[IBIS Ver]   3.2
[File Name]   sprm298.ibs
[File Rev]   1.0
[Date]   November 3, 2003
[Source]   File originated at Texas Instruments
[Copyright]   (c) 2003, Texas Instruments Inc.
[Component]   f2812pgf
[Manufacturer] Texas Instruments
[Package]
| Variable   Typ   Min   Max
R_pkg   0.198   0.1909   0.2047
L_pkg   8.904e-09   8.346e-09   9.905e-09
C_pkg   1.561e-12   1.156e-12   1.834e-12
[Pin] signal_name   model_name   R_pin   L_pin   C_pin
1   VDDAIO   NC   0.1921  9.905e-09  1.489e-12
2   ADCINB0   ioh125   0.1951  9.662e-09  1.834e-12
3   ADCINB1   ioh125   0.198   9.558e-09  1.805e-12
4   ADCINB2   ioh125   0.2006  9.473e-09  1.771e-12
5   ADCINB3   ioh125   0.2031  9.41e-09   1.706e-12
6   ADCINB4   ioh125   0.2036  9.308e-09  1.669e-12
7   ADCINB5   ioh125   0.2017  9.182e-09  1.673e-12
8   ADCINB6   ioh125   0.2002  9.071e-09  1.647e-12
9   ADCINB7   ioh125   0.1989  8.977e-09  1.625e-12
10   ADCREFM   ioh125   0.1977  8.88e-09   1.606e-12
11   ADCREFP   ioh125   0.1967  8.794e-09  1.581e-12
12   AVSSREFBG   ioh125   0.1961  8.721e-09  1.56e-12
13   AVDDREFBG   ioh125   0.1955  8.646e-09  1.544e-12
14   VDDA1   NC   0.195   8.579e-09  1.521e-12
15   VSSA1   NC   0.1949  8.524e-09  1.503e-12
16   ADCRESEXT   ioh125   0.1948  8.469e-09  1.489e-12
17   XMPNMC   idg095_pe1005   0.1948  8.424e-09  1.468e-12
18   XA(0)   oui835   0.1952  8.388e-09  1.452e-12
19   VSS   NC   0.1954  8.359e-09  1.442e-12
20   MDRA   idg095_ouo435_ps1005  0.196   8.346e-09  1.424e-12
21   XD(0)   idg095_oui835_ps1005  0.1967  8.36e-09   1.411e-12
22   MDXA   idg095_ouo435   0.1975  8.421e-09  1.16e-12
23   VDD   NC   0.198   8.429e-09  1.156e-12
24   XD(1)   idg095_oui835_ps1005  0.1973  8.376e-09  1.412e-12
25   MCLKRA   idg095_ouo435_ps1005  0.1971  8.373e-09  1.43e-12
26   MFSXA   idg095_ouo435_ps1005  0.197   8.398e-09  1.442e-12
27   XD(2)   idg095_oui835_ps1005  0.197   8.435e-09  1.457e-12
28   MCLKXA   idg095_ouo435_ps1005  0.1974  8.484e-09  1.476e-12
29   MFSRA   idg095_ouo435_ps1005  0.1977  8.542e-09  1.493e-12
30   XD(3)   idg095_oui835_ps1005  0.1984  8.61e-09   1.5e-12
31   VDDIO   NC   0.1982  8.656e-09  1.517e-12
32   VSS   NC   0.1989  8.731e-09  1.548e-12
33   XD(4)   idg095_oui835_ps1005  0.2001  8.817e-09  1.558e-12
34   SPICLKA   idg095_ouo435   0.1999  8.873e-09  1.577e-12
35   SPISTEA   idg095_ouo435   0.2013  8.967e-09  1.609e-12
36   XD(5)   idg095_oui835_ps1005  0.2027  9.071e-09  1.622e-12
37   VDD   NC   0.2027  9.139e-09  1.641e-12
38   VSS   NC   0.2047  9.255e-09  1.665e-12
39   XD(6)   idg095_oui835_ps1005  0.2047  9.341e-09  1.652e-12
40   SPISIMOA   idg095_ouo435   0.2031  9.409e-09  1.689e-12
41   SPISOMIA   idg095_ouo435   0.1983  9.422e-09  1.757e-12
42   XRDn   oui835   0.1956  9.501e-09  1.801e-12
43   XA(1)   oui835   0.1933  9.619e-09  1.832e-12
44   XZCS0AND1n   oui835   0.1909  9.876e-09  1.489e-12
45   PWM7   sw0145_ouo435_ups285  0.1921  9.905e-09  1.489e-12
46   PWM8   sw0145_ouo435_ups285  0.1951  9.662e-09  1.834e-12
47   PWM9   sw0145_ouo435_ups285  0.198   9.558e-09  1.805e-12
48   PWM10   sw0145_ouo435_ups285  0.2006  9.473e-09  1.771e-12
49   PWM11   sw0145_ouo435_ups285  0.2031  9.41e-09   1.706e-12
50   PWM12   sw0145_ouo435_ups285  0.2036  9.308e-09  1.669e-12
51   XRNW   oui835   0.2017  9.182e-09  1.673e-12
52   VSS   NC   0.2002  9.071e-09  1.647e-12
53   T3PWM_T3CMP   sw0145_ouo435_ups285  0.1989  8.977e-09  1.625e-12
54   XD(7)   idg095_oui835_ps1005  0.1977  8.88e-09   1.606e-12
55   T4PWM_T4CMP   sw0145_ouo435_ups285  0.1967  8.794e-09  1.581e-12
56   VDD   NC   0.1961  8.721e-09  1.56e-12
57   CAP4_QEP3   sw0145_ouo435_ups285  0.1955  8.646e-09  1.544e-12
58   VSS   NC   0.195   8.579e-09  1.521e-12
59   CAP5_QEP4   sw0145_ouo435_ups285  0.1949  8.524e-09  1.503e-12
60   CAP6_QEPI2   sw0145_ouo435_ups285  0.1948  8.469e-09  1.489e-12
61   C4TRIPn   sw0145_ouo435_ups285  0.1948  8.424e-09  1.468e-12
62   C5TRIPn   sw0145_ouo435_ups285  0.1952  8.388e-09  1.452e-12
63   C6TRIPn   sw0145_ouo435_ups285  0.1954  8.359e-09  1.442e-12
64   VDDIO   NC   0.196   8.346e-09  1.424e-12
65   XD(8)   idg095_oui835_ps1005  0.1967  8.36e-09   1.411e-12
66   TEST2   iog195   0.1975  8.421e-09  1.16e-12
67   TEST1   iog195   0.198   8.429e-09  1.156e-12
68   XD(9)   idg095_oui835_ps1005  0.1973  8.376e-09  1.412e-12
69   VDD3VFL   NC   0.1971  8.373e-09  1.43e-12
70   VSS   NC   0.197   8.398e-09  1.442e-12
71   TDIRB   sw0145_ouo435_ups285  0.197   8.435e-09  1.457e-12
72   TCLKINB   sw0145_ouo435_ups285  0.1974  8.484e-09  1.476e-12
73   XD(10)   idg095_oui835_ps1005  0.1977  8.542e-09  1.493e-12
74   XD(11)   idg095_oui835_ps1005  0.1984  8.61e-09   1.5e-12
75   VDD   NC   0.1982  8.656e-09  1.517e-12
76   X2   NC   0.1989  8.731e-09  1.548e-12
77   X1/XCLKIN   NC   0.2001  8.817e-09  1.558e-12
78   VSS   NC   0.1999  8.873e-09  1.577e-12
79   T3CTRIP_PDPINTBn idg095_ouo435_ps1005  0.2013  8.967e-09  1.609e-12
80   XA(2)   oui835   0.2027  9.071e-09  1.622e-12
81   VDDIO   NC   0.2027  9.139e-09  1.641e-12
82   XHOLDAn   oui835   0.2047  9.255e-09  1.665e-12
83   T4CTRIPn/EVBSOCn idg095_ouo435_ps1005  0.2047  9.341e-09  1.652e-12
84   XWEn   oui835   0.2031  9.409e-09  1.689e-12
85   XA(3)   oui835   0.1983  9.422e-09  1.757e-12
86   VSS   NC   0.1956  9.501e-09  1.801e-12
87   CANTXA   idg095_ouo435_ps1005  0.1933  9.619e-09  1.832e-12
88   XZCS2n   oui835   0.1909  9.876e-09  1.489e-12
89   CANRXA   idg095_ouo435_ps1005  0.1921  9.905e-09  1.489e-12
90   SCITXDB   idg095_ouo435   0.1951  9.662e-09  1.834e-12
91   SCIRXDB   idg095_ouo435   0.198   9.558e-09  1.805e-12
92   PWM1   idg095_ouo435_ps1005  0.2006  9.473e-09  1.771e-12
93   PWM2   idg095_ouo435_ps1005  0.2031  9.41e-09   1.706e-12
94   PWM3   idg095_ouo435_ps1005  0.2036  9.308e-09  1.669e-12
95   PWM4   idg095_ouo435_ps1005  0.2017  9.182e-09  1.673e-12
96   XD(12)   idg095_oui835_ps1005  0.2002  9.071e-09  1.647e-12
97   XD(13)   idg095_oui835_ps1005  0.1989  8.977e-09  1.625e-12
98   PWM5   idg095_ouo435_ps1005  0.1977  8.88e-09   1.606e-12
99   VSS   NC   0.1967  8.794e-09  1.581e-12
100   VDD   NC   0.1961  8.721e-09  1.56e-12
101   PWM6   idg095_ouo435_ps1005  0.1955  8.646e-09  1.544e-12
102   T1PWM_T1CMP   idg095_ouo435_ps1005  0.195   8.579e-09  1.521e-12
103   XA(4)   oui835   0.1949  8.524e-09  1.503e-12
104   T2PWM_T2CMP   idg095_ouo435_ps1005  0.1948  8.469e-09  1.489e-12
105   VSS   NC   0.1948  8.424e-09  1.468e-12
106   CAP1_QEP1   idg095_ouo435_ps1005  0.1952  8.388e-09  1.452e-12
107   CAP2_QEP2   idg095_ouo435_ps1005  0.1954  8.359e-09  1.442e-12
108   XA(5)   oui835   0.196   8.346e-09  1.424e-12
109   CAP3_QEPI1   idg095_ouo435_ps1005  0.1967  8.36e-09   1.411e-12
110   T1CTRIP_PDPINTAn idg095_ouo435_ps1005  0.1975  8.421e-09  1.16e-12
111   XA(6)   oui835   0.198   8.429e-09  1.156e-12
112   VDD   NC   0.1973  8.376e-09  1.412e-12
113   VSS   NC   0.1971  8.373e-09  1.43e-12
114   VDDIO   NC   0.197   8.398e-09  1.442e-12
115   T2CTRIPn/EVASOCn idg095_ouo435_ps1005  0.197   8.435e-09  1.457e-12
116   TDIRA   idg095_ouo435_ps1005  0.1974  8.484e-09  1.476e-12
117   TCLKINA   idg095_ouo435_ps1005  0.1977  8.542e-09  1.493e-12
118   XA(7)   oui835   0.1984  8.61e-09   1.5e-12
119   XCLKOUT   oui835   0.1982  8.656e-09  1.517e-12
120   VSS   NC   0.1989  8.731e-09  1.548e-12
121   XA(8)   oui835   0.2001  8.817e-09  1.558e-12
122   C1TRIPn   idg095_ouo435_ps1005  0.1999  8.873e-09  1.577e-12
123   C2TRIPn   idg095_ouo435_ps1005  0.2013  8.967e-09  1.609e-12
124   C3TRIPn   idg095_ouo435_ps1005  0.2027  9.071e-09  1.622e-12
125   XA(9)   oui835   0.2027  9.139e-09  1.641e-12
126   TMS   idg095_ps1005   0.2047  9.255e-09  1.665e-12
127   TDO   oui835   0.2047  9.341e-09  1.652e-12
128   VDD   NC   0.2031  9.409e-09  1.689e-12
129   VSS   NC   0.1983  9.422e-09  1.757e-12
130   XA(10)   oui835   0.1956  9.501e-09  1.801e-12
131   TDI   idg095_ps1005   0.1933  9.619e-09  1.832e-12
132   XA(11)   oui835   0.1909  9.876e-09  1.489e-12
133   XZCS6AND7n   oui835   0.1921  9.905e-09  1.489e-12
134   TESTSEL   idg095_pe1005   0.1951  9.662e-09  1.834e-12
135   TRSTn   idg095_pe1005   0.198   9.558e-09  1.805e-12
136   TCK   idg095_ps1005   0.2006  9.473e-09  1.771e-12
137   EMU0   idg095_oui835_ps1005  0.2031  9.41e-09   1.706e-12
138   XA(12)   oui835   0.2036  9.308e-09  1.669e-12
139   XD(14)   idg095_oui835_ps1005  0.2017  9.182e-09  1.673e-12
140   XF_XPLLDIS   idg095_oui835_ps1005  0.2002  9.071e-09  1.647e-12
141   XA(13)   oui835   0.1989  8.977e-09  1.625e-12
142   VSS   NC   0.1977  8.88e-09   1.606e-12
143   VDD   NC   0.1967  8.794e-09  1.581e-12
144   XA(14)   oui835   0.1961  8.721e-09  1.56e-12
145   VDDIO   NC   0.1955  8.646e-09  1.544e-12
146   EMU1   idg095_oui835_ps1005  0.195   8.579e-09  1.521e-12
147   XD(15)   idg095_oui835_ps1005  0.1949  8.524e-09  1.503e-12
148   XA(15)   oui835   0.1948  8.469e-09  1.489e-12
149   XINT1_XBIOn   idg095_ouo435   0.1948  8.424e-09  1.468e-12
150   XNMI_XINT13   idg095_ouo435_ps1005  0.1952  8.388e-09  1.452e-12
151   XINT2_ADCSOC   idg095_ouo435   0.1954  8.359e-09  1.442e-12
152   XA(16)   oui835   0.196   8.346e-09  1.424e-12
153   VSS   NC   0.1967  8.36e-09   1.411e-12
154   VDD   NC   0.1975  8.421e-09  1.16e-12
155   SCITXDA   idg095_ouo435_ps1005  0.198   8.429e-09  1.156e-12
156   XA(17)   oui835   0.1973  8.376e-09  1.412e-12
157   SCIRXDA   idg095_ouo435_ps1005  0.1971  8.373e-09  1.43e-12
158   XA(18)   oui835   0.197   8.398e-09  1.442e-12
159   XHOLDn   idg095_ps1005   0.197   8.435e-09  1.457e-12
160   XRSn   idg095_oum425_ps1005  0.1974  8.484e-09  1.476e-12
161   XREADY   idg095_ps1005   0.1977  8.542e-09  1.493e-12
162   VDD1   NC   0.1984  8.61e-09   1.5e-12
163   VSS1   NC   0.1982  8.656e-09  1.517e-12
164   ADCBGREFIN   ioh125   0.1989  8.731e-09  1.548e-12
165   VSSA2   NC   0.2001  8.817e-09  1.558e-12
166   VDDA2   NC   0.1999  8.873e-09  1.577e-12
167   ADCINA7   ioh125   0.2013  8.967e-09  1.609e-12
168   ADCINA6   ioh125   0.2027  9.071e-09  1.622e-12
169   ADCINA5   ioh125   0.2027  9.139e-09  1.641e-12
170   ADCINA4   ioh125   0.2047  9.255e-09  1.665e-12
171   ADCINA3   ioh125   0.2047  9.341e-09  1.652e-12
172   ADCINA2   ioh125   0.2031  9.409e-09  1.689e-12
173   ADCINA1   ioh125   0.1983  9.422e-09  1.757e-12
174   ADCINA0   ioh125   0.1956  9.501e-09  1.801e-12
175   ADCLO   ioh125   0.1933  9.619e-09  1.832e-12
176   VSSAIO   NC   0.1909  9.876e-09  1.489e-12
| End of package information
| Component idg095
[Component]   idg095
[Manufacturer]   Texas Instruments
[Package]
|   typ   min   max
R_pkg   0   0   0
L_pkg   0   0   0
C_pkg   0   0   0
[Pin]   signal_name   model_name   R_pin   L_pin   C_pin
   1   A   idg095   0   0   0
| Component idg095_oui835_ps1005
[Component]   idg095_oui835_ps1005
[Manufacturer]   Texas Instruments
[Package]
|   typ   min   max
R_pkg   0   0   0
L_pkg   0   0   0
C_pkg   0   0   0
[Pin]   signal_name   model_name   R_pin   L_pin   C_pin
   1   Y  idg095_oui835_ps1005   0   0   0
| Component idg095_oum425_ps1005
[Component]   idg095_oum425_ps1005
[Manufacturer]   Texas Instruments
[Package]
|   typ   min   max
R_pkg   0   0   0
L_pkg   0   0   0
C_pkg   0   0   0
[Pin]   signal_name   model_name   R_pin   L_pin   C_pin
   1   Y  idg095_oum425_ps1005   0   0   0
| Component idg095_ouo435_ps1005
[Component]   idg095_ouo435_ps1005
[Manufacturer]   Texas Instruments
[Package]
|   typ   min   max
R_pkg   0   0   0
L_pkg   0   0   0
C_pkg   0   0   0
[Pin]   signal_name   model_name   R_pin   L_pin   C_pin
   1   Y  idg095_ouo435_ps1005   0   0   0
| Component idg095_pe1005
[Component]   idg095_pe1005
[Manufacturer]   Texas Instruments
[Package]
|   typ   min   max
R_pkg   0   0   0
L_pkg   0   0   0
C_pkg   0   0   0
[Pin]   signal_name   model_name   R_pin   L_pin   C_pin
   1   A   idg095_pe1005   0   0   0
| Component idg095_ps1005
[Component]   idg095_ps1005
[Manufacturer]   Texas Instruments
[Package]
|   typ   min   max
R_pkg   0   0   0
L_pkg   0   0   0
C_pkg   0   0   0
[Pin]   signal_name   model_name   R_pin   L_pin   C_pin
   1   A   idg095_ps1005   0   0   0
| Component iog195
[Component]   iog195
[Manufacturer]   Texas Instruments
[Package]
|   typ   min   max
R_pkg   0   0   0
L_pkg   0   0   0
C_pkg   0   0   0
[Pin]   signal_name   model_name   R_pin   L_pin   C_pin
   1   Y   iog195   0   0   0
| Component ioh125
[Component]   ioh125
[Manufacturer]   Texas Instruments
[Package]
|   typ   min   max
R_pkg   0   0   0
L_pkg   0   0   0
C_pkg   0   0   0
[Pin]   signal_name   model_name   R_pin   L_pin   C_pin
   1   Y   ioh125   0   0   0
| Component oui835
[Component]   oui835
[Manufacturer]   Texas Instruments
[Package]
|   typ   min   max
R_pkg   0   0   0
L_pkg   0   0   0
C_pkg   0   0   0
[Pin]   signal_name   model_name   R_pin   L_pin   C_pin
   1   Y   oui835   0   0   0
| Component oum425
[Component]   oum425
[Manufacturer]   Texas Instruments
[Package]
|   typ   min   max
R_pkg   0   0   0
L_pkg   0   0   0
C_pkg   0   0   0
[Pin]   signal_name   model_name   R_pin   L_pin   C_pin
   1   Y   oum425   0   0   0
| Component idg095_ouo435
[Component]   idg095_ouo435
[Manufacturer]   Texas Instruments
[Package]
|   typ   min   max
R_pkg   0   0   0
L_pkg   0   0   0
C_pkg   0   0   0
[Pin]   signal_name   model_name   R_pin   L_pin   C_pin
   1   Y   idg095_ouo435   0   0   0
| Component ouo435
[Component]   ouo435
[Manufacturer]   Texas Instruments
[Package]
|   typ   min   max
R_pkg   0   0   0
L_pkg   0   0   0
C_pkg   0   0   0
[Pin]   signal_name   model_name   R_pin   L_pin   C_pin
   1   Y   ouo435   0   0   0
| Component sw0145_ouo435_ups285
[Component]   sw0145_ouo435_ups285
[Manufacturer]   Texas Instruments
[Package]
|   typ   min   max
R_pkg   0   0   0
L_pkg   0   0   0
C_pkg   0   0   0
[Pin]   signal_name   model_name   R_pin   L_pin   C_pin
   1   Y  sw0145_ouo435_ups285   0   0   0
| Models and submodels in the file (13): idg095 (Input), idg095_oui835_ps1005 (I/O), idg095_oum425_ps1005 (I/O_open_sink), idg095_ouo435_ps1005 (I/O), idg095_pe1005 (Input), idg095_ps1005 (Input), iog195 (Terminator), ioh125 (Terminator), oui835 (3-state), oum425 (I/O_open_sink), idg095_ouo435 (I/O), ouo435 (3-state), sw0145_ouo435_ups285 (I/O)
